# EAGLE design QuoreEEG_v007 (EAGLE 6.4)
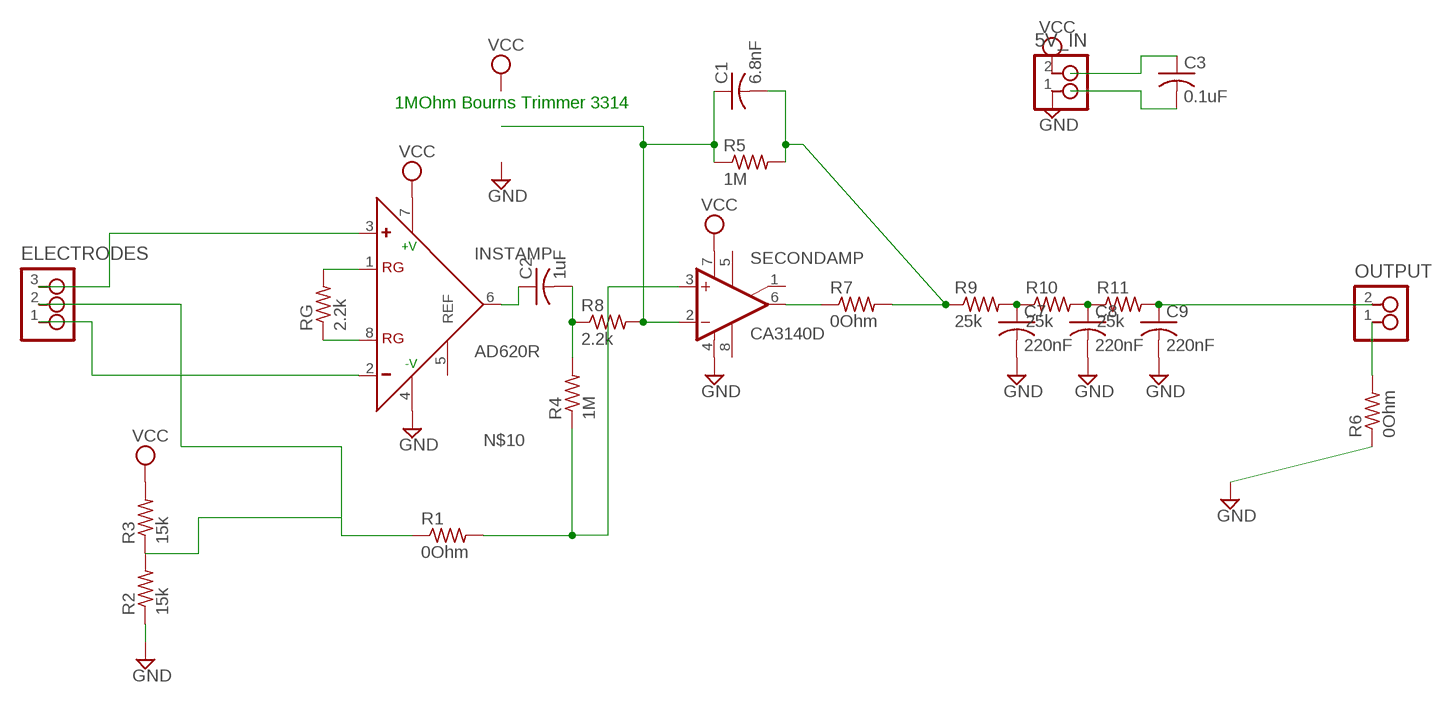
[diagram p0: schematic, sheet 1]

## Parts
5V_IN  2_PIN_HEADERHEADER  [SMT_PINS_2]
C1  6.8nF  C-USC1206  [C1206]
C2  1uF  C-USC1206  [C1206]
C3  0.1uF  C-USC1206  [C1206]
C7  220nF  C-USC1206  [C1206]
C8  220nF  C-USC1206  [C1206]
C9  220nF  C-USC1206  [C1206]
ELECTRODES  3_PIN_HEADERHEADER  [SMT_PINS_3]
INSTAMP  AD620R  [SO8]
OUTPUT  2_PIN_HEADERHEADER  [SMT_PINS_2]
R1  0Ohm  R-US_R1206  [R1206]
R2  15k  R-US_R1206  [R1206]
R3  15k  R-US_R1206  [R1206]
R4  1M  R-US_R1206  [R1206]
R5  1M  R-US_R1206  [R1206]
R6  0Ohm  R-US_R1206  [R1206]
R7  0Ohm  R-US_R1206  [R1206]
R8  2.2k  R-US_R1206  [R1206]
R9  25k  R-US_R1206  [R1206]
R10  25k  R-US_R1206  [R1206]
R11  25k  R-US_R1206  [R1206]
RG  2.2k  R-US_R1206  [R1206]
SECONDAMP  CA3140D  [SO08]

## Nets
GND: 5V_IN.1 C7.2 C8.2 C9.2 INSTAMP.4(-V) R2.1 R6.1 SECONDAMP.4(V-)
N$1: INSTAMP.1(RG) RG.2
N$2: INSTAMP.8(RG) RG.1
N$3: ELECTRODES.3 INSTAMP.3(+)
N$4: C1.2 R5.2 R7.2 R9.1
N$5: C1.1 R5.1 R8.2 SECONDAMP.2(-IN)
N$8: C2.1 INSTAMP.6(OUT)
N$9: C2.2 R4.2 R8.1
N$10: R1.2 R4.1 SECONDAMP.3(+IN)
N$12: C7.1 R9.2 R10.1
N$15: ELECTRODES.1 INSTAMP.2(-)
N$17: OUTPUT.1 R6.2
N$18: R7.1 SECONDAMP.6(OUT)
N$20: C8.1 R10.2 R11.1
N$21: C3.1
N$22: C3.2
N$25: C9.1 OUTPUT.2 R11.2
VCC: 5V_IN.2 INSTAMP.7(+V) R3.2 SECONDAMP.7(V+)
VIRT_GND: ELECTRODES.2 R1.1 R2.2 R3.1
Unconnected: INSTAMP.5(REF) SECONDAMP.1(ON/CMP) SECONDAMP.5(ON) SECONDAMP.8(CMP)

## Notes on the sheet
- 1MOhm Bourns Trimmer 3314

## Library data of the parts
5V_IN OUTPUT = ng:2_PIN_HEADER: 2 SMT pin pads
C1 C2 C7-C9 = rcl:C-US: CAPACITOR, American symbol
C3 = resistor:C-US: CAPACITOR, American symbol
ELECTRODES = ng:3_PIN_HEADER: 3 SMT pin pads
INSTAMP = analog-devices:AD620: Low Cost, Low Power, Instrumentation Amplifier Source: http://www.analog.com/UploadedFiles/Data_Sheets/37793330023930AD620_e.pdf
R1-R11 RG = resistor:R-US_: RESISTOR, American symbol
SECONDAMP = linear:CA3140: OP AMP

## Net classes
0 default: drill 0.813 mm

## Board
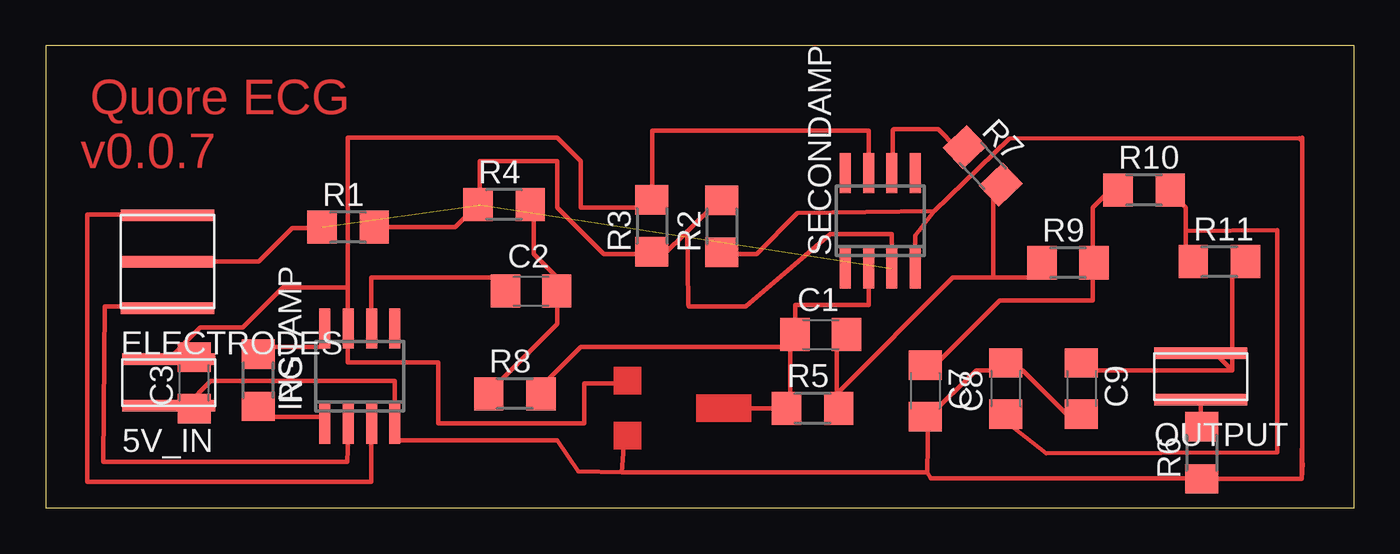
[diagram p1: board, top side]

Size 71.38 x 25.23 mm. Coordinates in mm from the lower left corner, seen from the top.
Outline: 0,0 71.38,0 71.38,25.23 0,25.23 0,0
Copper layers (1*16): Top 0.035mm / dielectric 1.5mm / Bottom 0.035mm
Design rules "default": minimum track width 12mil, minimum drill 0.8mm, track to track 15.5mil, track to pad 15.5mil, pad to pad 15mil, via to via 15mil, smd to smd 10mil, copper to edge 0mil, drill to drill 1mm, minimum pad ring 0.2mm, minimum via ring 0.2mm, stop-mask expansion 4mil, vias tented up to drill 0mil, thermal gap 1mm

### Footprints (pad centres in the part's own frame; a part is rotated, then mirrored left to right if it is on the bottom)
SMT_PINS_2 = smd 5.08 x 0.635: 1 0,0; 2 0,2.54
C1206 = smd 1.6 x 1.8: 1 -1.4,0; 2 1.4,0
SMT_PINS_3 = smd 5.08 x 0.635: 1 0,0; 2 0,2.54; 3 0,5.08
SO8 = smd 0.6 x 2.2: 1 -1.905,-2.6; 2 -0.635,-2.6; 3 0.635,-2.6; 4 1.905,-2.6; 5 1.905,2.6; 6 0.635,2.6; 7 -0.635,2.6; 8 -1.905,2.6
R1206 = smd 1.6 x 1.803: 1 -1.422,0; 2 1.422,0
SO08 = smd 0.6 x 2.2: 1 -1.905,-2.6; 2 -0.635,-2.6; 3 0.635,-2.6; 4 1.905,-2.6; 5 1.905,2.6; 6 0.635,2.6; 7 -0.635,2.6; 8 -1.905,2.6

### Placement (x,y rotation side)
5V_IN  6.7,5.57 0 top
C1  42.27,9.45 0 top
C2  26.47,11.83 0 top
C3  8.09,6.81 90 top
C7  47.98,6.38 270 top
C8  52.38,6.51 90 top
C9  56.5,6.51 270 top
ELECTRODES  6.64,10.9 0 top
INSTAMP  17.13,7.19 0 top
OUTPUT  63.01,5.9 0 top
R1  16.5,15.32 0 top
R2  36.87,15.37 90 top
R3  33.07,15.39 90 top
R4  25,16.55 0 top
R5  41.84,5.43 0 top
R6  63.06,3 90 top
R7  51.12,18.67 313.6 top
R8  25.59,6.23 0 top
R9  55.77,13.38 0 top
R10  59.92,17.35 0 top
R11  64.02,13.43 0 top
RG  11.59,6.96 270 top
SECONDAMP  45.52,15.67 0 top

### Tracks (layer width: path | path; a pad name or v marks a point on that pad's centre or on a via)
GND
  Top 0.254: 48.15,4.96 50.76,7.5 52.03,7.5 | 52.03,7.5 53.3,7.5 55.84,4.96 C9.2 | 52.03,7.5 C8.2 | 68.54,20.02 68.54,2.42 68.57,2.42 68.52,1.58 | 68.54,20.02 68.54,20.2 | 48.15,4.96 48.09,1.94 | 48.09,1.94 48.27,1.61 63.11,1.61 R6.1 68.52,1.58 | R2.1 36.79,13.85 38.77,13.85 41.01,16.08 48.48,16.21 | 48.15,4.96 C7.2 | 48.09,1.94 31.43,1.94 | 31.43,1.94 29.04,1.99 27.9,3.69 19.01,3.69 INSTAMP.4 19.04,6.91 9,6.91 7.66,5.57 5V_IN.1 | 48.48,16.21 52.56,20.15 68.39,20.17 68.54,20.02 | SECONDAMP.4 47.43,14.86 48.48,16.21 | 31.56,3.71 31.43,1.94 | 68.52,1.58 68.52,3.21
N$1
  Top 0.254: RG.2 11.39,4.96 15.2,4.96 INSTAMP.1
N$2
  Top 0.254: RG.1 11.39,8.77 15.2,8.77 INSTAMP.8
N$3
  Top 0.254: INSTAMP.3 17.77,1.4 2.27,1.4 2.27,16.01 6.64,16.01 ELECTRODES.3
N$4
  Top 0.254: 43.14,6.23 43.14,8.77 C1.2 | 51.68,12.58 49.49,12.58 43.14,6.23 | 51.68,12.58 54.57,12.58 R9.1 | 43.14,6.23 R5.2 | R7.2 51.68,17.22 51.68,12.58
N$5
  Top 0.254: 40.6,8.77 40.6,6.23 R5.1 | 40.6,8.77 29.17,8.77 26.63,6.23 R8.2 | 40.6,8.77 C1.1 40.88,11.08 44.89,11.08 SECONDAMP.2
N$6
  Top 0.254: 16.52,9.71 16.47,9.71 16.47,7.93 21.4,7.93 21.4,4.6 29.37,4.6 29.37,6.79 31.56,6.79
N$8
  Top 0.254: C2.1 25.36,12.58 17.74,12.58 17.74,10.04 INSTAMP.6
N$9
  Top 0.254: R4.2 26.63,16.39 26.63,13.85 27.9,12.58 C2.2 27.9,11.31 27.9,10.04 24.09,6.23 R8.1
N$10  (1 unrouted)
  Top 0.254: R1.2 22.35,15.32 R4.1
N$12
  Top 0.254: C7.1 48.22,7.5 52.03,11.31 57.11,11.31 57.11,12.58 R9.2 57.11,13.85 57.11,16.39 58.38,17.66 R10.1
N$15
  Top 0.254: INSTAMP.2 16.52,4.59 16.45,2.52 3.14,2.52 3.21,11 6.82,11 ELECTRODES.1
N$17
  Top 0.254: R6.2 63.01,4.42 OUTPUT.1
N$18
  Top 0.254: SECONDAMP.6 46.21,18.27 46.21,20.63 46.27,20.68 48.68,20.68 49.66,19.7 R7.1
N$19
  Top 0.254: 38.14,5.42 40.22,5.42
N$20
  Top 0.254: 62.19,15.12 67.17,15.17 67.17,3.03 54.57,2.98 52.03,4.96 C8.1 | 62.19,15.12 62.19,13.85 R11.1 | 62.19,15.12 62.19,16.39 60.92,17.66 R10.2
N$25
  Top 0.254: 64.73,7.5 57.11,7.5 C9.1 | 64.73,7.5 64.73,12.58 R11.2 | 64.73,7.5 63.79,8.44 OUTPUT.2
VCC
  Top 0.254: 16.47,12.02 16.47,10.04 INSTAMP.7 | 16.47,12.02 16.47,20.2 27.9,20.2 29.17,18.93 29.17,16.39 32.98,16.39 R3.2 33.08,16.82 33.08,20.58 44.89,20.58 SECONDAMP.7 | 5V_IN.2 8.42,9.84 10.73,9.84 12.92,12.02 16.47,12.02
VIRT_GND  (1 unrouted)
  Top 0.254: 32.98,13.85 30.44,13.85 27.9,16.39 27.9,18.93 23.69,18.93 23.69,16.54 | 34.99,15.09 33.69,13.8 32.98,13.85 | 34.99,15.09 36.74,16.79 R2.2 | 32.98,13.85 R3.1 | 34.99,15.09 35.04,11.13 35.06,11 38.19,11 42.79,14.94 46.16,14.94 46.16,13.07 | ELECTRODES.2 11.61,13.44 13.45,15.27 15.02,15.27 R1.1
(copper drawn outside any net)
  shapes: Top area x3

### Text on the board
Top: Quore ECG | v0.0.7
